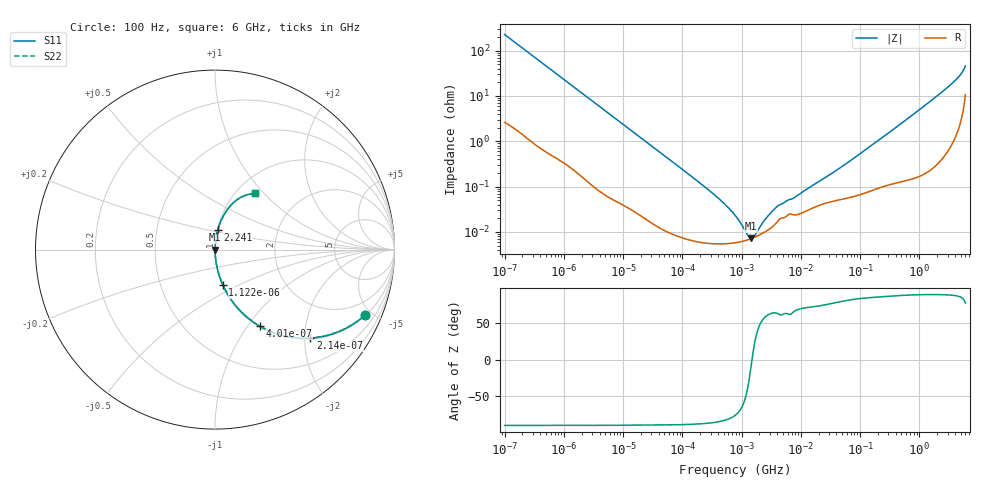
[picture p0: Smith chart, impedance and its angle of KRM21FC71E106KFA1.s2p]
!Murata Part Number: KRM21FC71E106KFA1
!These Parameters are Measured in Series Mode Connection
!Data Generated on Jan 08, 2026
!  o--ll--o
!Port1  Port2
!  o------o
!Operation Temp=25[degC], DC Bias Voltage=0[V]
!Freq. Start=100[Hz] Stop=6[GHz] 401[Steps]
# Hz S RI R 50
!Freq.(Hz) S11(Real) S11(Imag) S21(Real) S21(Imag) S12(Real) S12(Imag) S22(Real) S22(Imag)
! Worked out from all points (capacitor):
!   401 points, 100 Hz to 6 GHz, reference 50 ohm
!   read as one part in series: C = 7 uF near 109 Hz
!   lowest |Z| = 7.17 mohm at 1.45 MHz (marker M1)
!   series resonance near 1.5 MHz, so ESL is about 1.6 nH
!   S11 on the Smith chart (normalised r, x): 100 Hz: 1.05, -4.53; 214 Hz: 1.03, -2.13; 401 Hz: 1.01, -1.14; 1.122 kHz: 1.01, -0.41; 2.241 GHz: 1.01, +0.23; 6 GHz: 1.21, +0.89
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100  0.8343 -0.3661  0.1657 0.3661  0.1657 0.3661  0.8343 -0.3661
214  0.5319 -0.4929  0.4681 0.4929  0.4681 0.4929  0.5319 -0.4929
401  0.2495 -0.4267  0.7505 0.4267  0.7505 0.4267  0.2495 -0.4267
627  0.122 -0.3207  0.878 0.3207  0.878 0.3207  0.122 -0.3207
1122  0.0434 -0.1967  0.9566 0.1967  0.9566 0.1967  0.0434 -0.1967
2008  0.0148 -0.114  0.9852 0.114  0.9852 0.114  0.0148 -0.114
6433  0.00186 -0.0364  0.9981 0.0364  0.9981 0.0364  0.00186 -0.0364
40335  0.000159 -0.00593  0.9998 0.00593  0.9998 0.00593  0.000159 -0.00593
330837  5.53e-05 -0.000695  0.9999 0.000695  0.9999 0.000695  5.53e-05 -0.000695
774597  5.74e-05 -0.000227  0.9999 0.000227  0.9999 0.000227  5.74e-05 -0.000227
1159002  6.43e-05 -8.22e-05  0.9999 8.22e-05  0.9999 8.22e-05  6.43e-05 -8.22e-05
1449809  7.09e-05 -1.06e-05  0.9999 1.06e-05  0.9999 1.06e-05  7.09e-05 -1.06e-05
1813585  8.04e-05 5.87e-05  0.9999 -5.87e-05  0.9999 -5.87e-05  8.04e-05 5.87e-05
2713602  0.000107 0.000187  0.9999 -0.000187  0.9999 -0.000187  0.000107 0.000187
4060267  0.000172 0.000329  0.9998 -0.000329  0.9998 -0.000329  0.000172 0.000329
7599586  0.000237 0.000507  0.9998 -0.000507  0.9998 -0.000507  0.000237 0.000507
1.555665e7  0.000333 0.000994  0.9997 -0.000994  0.9997 -0.000994  0.000333 0.000994
4.983056e7  0.000532 0.00272  0.9995 -0.00272  0.9995 -0.00272  0.000532 0.00272
3.124326e8  0.00134 0.0157  0.9987 -0.0157  0.9987 -0.0157  0.00134 0.0157
2.240541e9  0.016 0.1105  0.984 -0.1105  0.984 -0.1105  0.016 0.1105
4.385646e9  0.0693 0.224  0.9307 -0.224  0.9307 -0.224  0.0693 0.224
6e9  0.2216 0.3134  0.7784 -0.3134  0.7784 -0.3134  0.2216 0.3134
